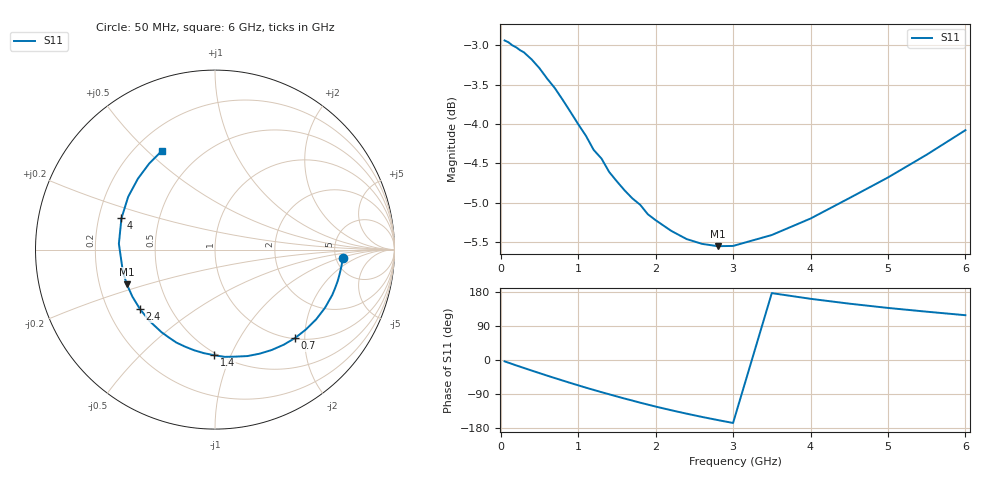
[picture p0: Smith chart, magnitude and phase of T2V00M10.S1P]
! SIEMENS Discrete & RF Semiconductors
! BAS70-04W
! Si Schottky Diode in SOT323
! IF = 0.1 mA
! S-Parameters:  November  1997
# GHz  S  MA  R  50
!  f  S11
! GHz  MAG  ANG
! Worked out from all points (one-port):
!   34 points, 50 MHz to 6 GHz, reference 50 ohm
!   lowest |S11| = -5.5 dB at 2.8 GHz (marker M1), VSWR 3.24, Z = 16 - j8.6 ohm
!   |S11| at or under -10 dB: nowhere
!   S11 on the Smith chart (normalised r, x): 50 MHz: 5.77, -1.05; 700 MHz: 1.02, -1.79; 1.4 GHz: 0.48, -0.87; 2.4 GHz: 0.34, -0.31; 4 GHz: 0.30, +0.15; 6 GHz: 0.31, +0.56
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0.05  0.7129 -3.6
0.15  0.7078 -10.7
0.2  0.7058 -14.3
0.3  0.7006 -21.1
0.4  0.6934 -27.9
0.5  0.6846 -34.6
0.6  0.6742 -41.3
0.7  0.6649 -47.8
0.8  0.6537 -54.2
0.9  0.6423 -60.6
1  0.6309 -66.8
1.1  0.6202 -73.0
1.3  0.6 -84.8
1.4  0.5883 -90.5
1.6  0.5726 -101.8
1.8  0.5608 -112.6
2  0.5483 -122.9
2.2  0.5399 -132.5
2.4  0.5334 -141.6
2.6  0.5296 -150.3
2.8  0.5279 -158.4
3  0.528 -166.2
3.5  0.5365 176.5
4  0.5496 161.5
4.5  0.5662 148.7
5  0.5836 137.4
5.5  0.6033 127.5
6  0.6253 118.2
